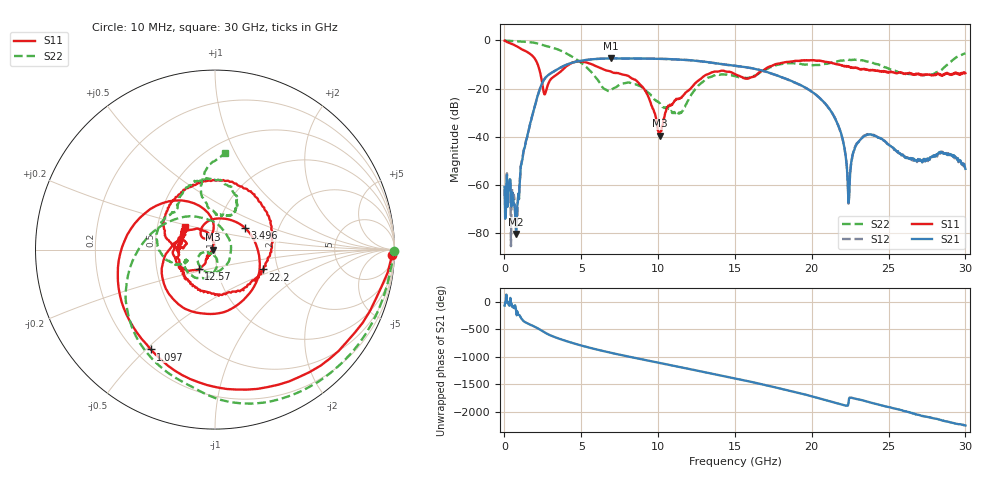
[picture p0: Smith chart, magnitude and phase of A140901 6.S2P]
!  2-Port S-parameters saved by WinCal
! VAR MeasName=S-Parameters (CALIBRATED_DATA) read from VNA (N5244A)
! VAR MeasDate=11/3/2014 9:27:02 AM
! VAR NAME=A140901 6
! VAR FILENAME=A140901 6.S2P
! VAR DATE=11/3/2014 9:27:02 AM
! VAR PHYS_PORTS=1,2
# Hz S RI R 50
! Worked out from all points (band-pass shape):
!   801 points, 10 MHz to 30 GHz, reference 50 ohm
!   highest |S21| = -7.44 dB at 6.908 GHz (marker M1); lowest = -80.2 dB at 759.8 MHz (marker M2)
!   |S21| within 3 dB of the highest: 3.909 GHz to 14.89 GHz (10.98 GHz wide, 117 % of centre)
!   lowest |S11| = -39.5 dB at 10.09 GHz (marker M3), VSWR 1.02, Z = 49 - j0.112 ohm
!   |S11| at or under -10 dB: 2.168 GHz to 4.211 GHz (2.043 GHz wide, 64.1 % of centre); 5.73 GHz to 17.58 GHz (11.85 GHz wide, 102 % of centre); 21.76 GHz to end of sweep
!   |S22| runs from -30.3 to 0.0 dB; largest |S21 - S12| = 0.0037
!   S11 on the Smith chart (normalised r, x): 10 MHz: 22, -54; 1.097 GHz: 0.26, -0.52; 3.496 GHz: 1.36, +0.34; 12.57 GHz: 0.82, -0.18; 22.2 GHz: 1.67, -0.40; 30 GHz: 0.69, +0.19
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1e7  0.9865 -0.0316  0.000318 -0.000868  -0.000786 0.000162  0.9975 -0.00807
7.5975e8  0.0105 -0.7675  -9.2e-05 -3.4e-05  -0.000272 -7.86e-05  0.8496 -0.4534
1.097138e9  -0.3578 -0.5564  0.0016 0.00222  0.00166 0.00223  0.7232 -0.6149
2.334225e9  -0.0388 0.2046  -0.0914 -0.0516  -0.0912 -0.0517  0.00976 -0.8303
2.634125e9  -0.0435 0.0632  -0.1523 0.0589  -0.1518 0.0586  -0.1358 -0.7605
3.496338e9  0.168 0.1198  0.1504 0.2085  0.1501 0.2088  -0.4485 -0.4654
5.033325e9  -0.2041 -0.304  0.0744 -0.3744  0.0741 -0.3749  -0.3136 0.1224
6.9077e9  -0.2236 0.0376  -0.3783 0.1929  -0.3778 0.1937  0.0852 -0.0323
8.969512e9  -0.0474 0.0998  0.3575 0.2216  0.3564 0.2217  -0.0951 -0.0453
1.001916e10  -0.0123 0.00447  0.3687 -0.196  0.3683 -0.1952  -0.0514 -0.0146
1.009414e10  -0.0106 -0.00114  0.3521 -0.2225  0.3517 -0.2222  -0.0476 -0.015
1.144369e10  -0.0434 -0.0459  -0.1297 -0.3776  -0.1294 -0.3777  -0.00807 -0.03
1.256831e10  -0.0904 -0.11  -0.3727 -0.0415  -0.3721 -0.0411  0.0029 -0.11
1.5005e10  -0.1937 0.0504  0.2007 0.2202  0.2009 0.2178  -0.1675 -0.0696
1.695435e10  -0.2501 0.0426  0.0646 -0.2174  0.0651 -0.2164  -0.2294 -0.0803
2.002832e10  0.0728 0.3837  0.0144 0.0843  0.0138 0.0844  -0.2195 0.2113
2.152782e10  0.32 0.0721  0.0196 -0.014  0.0198 -0.0138  -0.1883 0.3042
2.22026e10  0.2679 -0.1108  0.000139 -0.00416  0.000169 -0.00418  -0.1246 0.3691
2.242752e10  0.2428 -0.1565  0.000394 0.000325  0.000388 0.000493  -0.1015 0.3821
2.328974e10  0.0498 -0.2459  0.00938 0.0017  0.00965 0.00182  0.029 0.3876
2.501416e10  -0.1838 -0.1133  -0.00282 -0.00618  -0.00281 -0.00639  0.1181 0.2339
3e10  -0.1662 0.1275  7.52e-05 -0.00218  -2.9e-05 -0.00241  0.0567 0.5385
